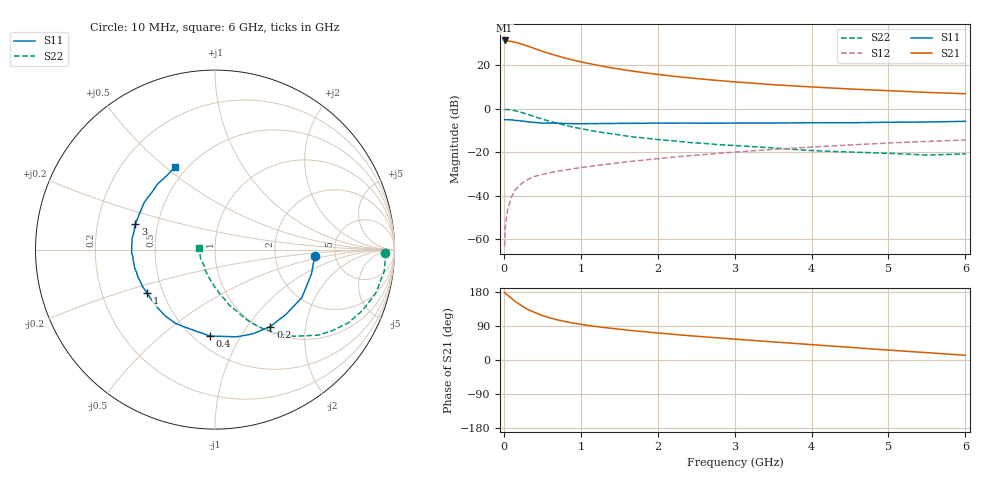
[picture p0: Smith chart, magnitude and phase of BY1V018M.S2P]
! SIEMENS Small Signal Semiconductors
! BFY420
! Si NPN RF SIEGET Grounded Emitter Transistor in MICRO-X
! VCE = 1 V  IC = 18 mA
! Common Emitter S-Parameters:  October  1996
# GHz  S  MA  R  50
!  f  S11  S21  S12  S22
! GHz  MAG  ANG  MAG  ANG  MAG  ANG  MAG  ANG
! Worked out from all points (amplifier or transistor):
!   36 points, 10 MHz to 6 GHz, reference 50 ohm
!   highest |S21| = 31.3 dB at 10 MHz (marker M1)
!   |S21| within 3 dB of that: start of sweep to 342.9 MHz
!   unconditionally stable (mu >= 1): start of sweep to 10.72 MHz; 1.917 GHz to end of sweep
!   at 250 MHz: K = 0.28, MSG = 31.6 dB, |S12| = -33.9 dB
!   at 1.4 GHz: K = 0.91, MSG = 22.0 dB, |S12| = -25.3 dB
!   at 6 GHz: K = 1.10, MAG = 8.7 dB, |S12| = -14.4 dB
!   S11 on the Smith chart (normalised r, x): 10 MHz: 3.50, -0.34; 200 MHz: 1.09, -1.30; 400 MHz: 0.60, -0.75; 1 GHz: 0.41, -0.25; 3 GHz: 0.37, +0.14; 6 GHz: 0.43, +0.54
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0.01  0.5587 -3.4  36.54 178.9  0.0007 110.2  0.9493 -1.0
0.02  0.5545 -6.4  36.31 175.8  0.0021 92.6  0.9505 -2.6
0.1  0.5529 -28.9  34.67 162.9  0.0095 79.7  0.9279 -15.2
0.15  0.5354 -42.1  33.05 154.1  0.0137 73.7  0.8892 -22.4
0.2  0.5283 -54.3  31.41 147.5  0.0172 69.7  0.848 -28.7
0.25  0.5142 -66.1  29.38 140.4  0.0203 65.9  0.7956 -34.5
0.3  0.5008 -76.0  27.48 134.7  0.023 63.0  0.749 -39.5
0.4  0.4823 -93.3  23.87 125.5  0.0278 57.3  0.6532 -47.7
0.5  0.464 -107.2  20.57 117.3  0.031 55.0  0.5737 -54.0
0.6  0.4666 -118.4  18.16 111.1  0.0338 53.9  0.51 -59.1
0.7  0.4615 -127.6  16.14 105.8  0.0367 53.3  0.4579 -63.4
0.8  0.4551 -135.1  14.36 101.4  0.039 51.9  0.4126 -66.9
1  0.4486 -147.3  11.82 94.2  0.0442 52.4  0.3476 -72.2
1.1  0.453 -152.4  10.87 91.1  0.0468 52.5  0.3224 -75.2
1.4  0.4549 -163.8  8.582 83.5  0.0543 52.7  0.265 -81.4
1.6  0.4587 -170.0  7.548 78.9  0.0601 52.4  0.2349 -85.6
2.2  0.4644 176.0  5.525 67.8  0.0769 50.9  0.1827 -95.9
3  0.4659 162.0  4.105 55.1  0.1007 47.1  0.1426 -107.7
3.5  0.4666 153.7  3.537 47.8  0.1158 43.8  0.1253 -116.1
4.5  0.4742 138.7  2.818 33.4  0.1467 35.3  0.1009 -132.6
5.5  0.4927 122.8  2.351 19.4  0.1769 25.8  0.0861 -166.3
6  0.5107 115.9  2.194 12.4  0.1907 20.8  0.0912 174.4
